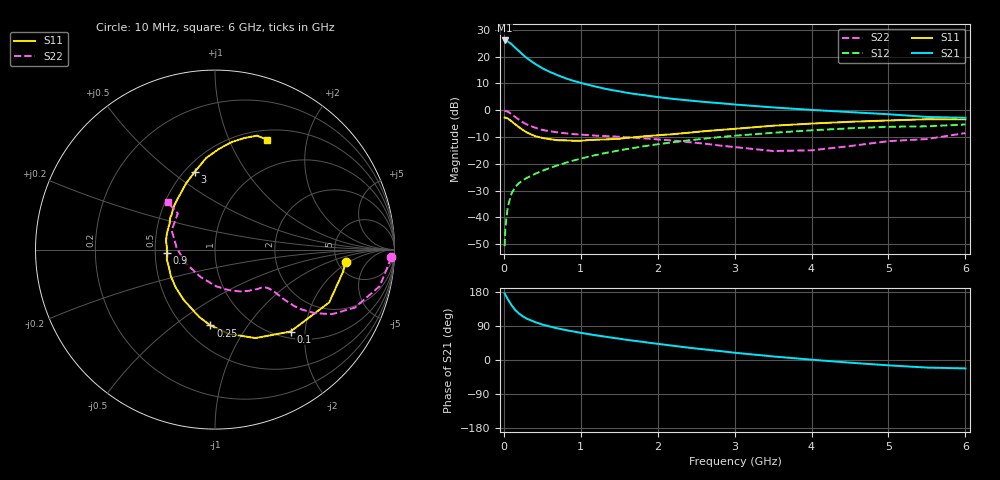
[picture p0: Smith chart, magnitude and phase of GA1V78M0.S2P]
! Infineon Technologies  Discrete & RF Semiconductors
! BF775
! Si NPN RF Bipolar Junction Transistor in SOT23
! VCE = 1.75 V  IC = 8 mA
! Common Emitter S-Parameters:  May  1996
# GHz  S  MA  R  50
!  f  S11  S21  S12  S22
! GHz  MAG  ANG  MAG  ANG  MAG  ANG  MAG  ANG
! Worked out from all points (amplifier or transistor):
!   36 points, 10 MHz to 6 GHz, reference 50 ohm
!   highest |S21| = 26.0 dB at 10 MHz (marker M1)
!   |S21| within 3 dB of that: start of sweep to 159.2 MHz
!   unconditionally stable (mu >= 1): 594.3 MHz to 3.973 GHz; 5.424 GHz to 5.631 GHz
!   at 250 MHz: K = 0.64, MSG = 23.4 dB, |S12| = -26.1 dB
!   at 1.4 GHz: K = 1.14, MAG = 9.3 dB, |S12| = -15.6 dB
!   at 6 GHz: K = 0.99, MSG = 1.2 dB, |S12| = -5.3 dB
!   S11 on the Smith chart (normalised r, x): 10 MHz: 5.91, -1.71; 100 MHz: 1.13, -1.68; 250 MHz: 0.67, -0.69; 900 MHz: 0.58, -0.02; 3 GHz: 0.56, +0.61; 6 GHz: 0.62, +1.39
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0.01  0.7304 -5.3  19.97 176.1  0.0029 86.4  0.982 -2.5
0.02  0.7239 -9.9  19.63 172.0  0.0063 85.8  0.9694 -5.1
0.05  0.701 -24.8  19.18 160.9  0.0155 77.0  0.9404 -12.5
0.1  0.6211 -47.3  17.06 144.6  0.0279 68.8  0.8436 -22.5
0.15  0.5421 -65.4  14.53 131.5  0.0371 63.0  0.7446 -28.9
0.2  0.4765 -80.5  12.54 122.1  0.044 60.3  0.6588 -32.5
0.25  0.4236 -93.4  10.74 114.7  0.0494 58.1  0.5896 -34.6
0.3  0.385 -103.3  9.346 109.0  0.0547 58.3  0.5416 -35.5
0.4  0.3293 -122.3  7.411 100.6  0.0642 58.2  0.4735 -35.8
0.5  0.3036 -136.3  6.066 93.7  0.0738 59.2  0.4288 -35.5
0.6  0.2872 -149.0  5.152 88.2  0.0838 59.7  0.4031 -35.4
0.7  0.275 -159.1  4.487 83.5  0.0934 60.4  0.3853 -35.6
0.9  0.2686 -176.1  3.546 75.4  0.1143 60.8  0.3589 -36.3
1.1  0.277 170.1  2.965 68.4  0.1353 60.2  0.3423 -38.3
1.3  0.2835 159.4  2.539 62.1  0.1567 59.2  0.3292 -40.8
1.6  0.3058 144.6  2.111 53.2  0.1882 56.8  0.3109 -45.9
2.2  0.3562 124.6  1.621 37.6  0.2519 51.0  0.2712 -59.3
3  0.4483 104.5  1.276 19.2  0.3333 41.2  0.2048 -88.0
3.5  0.5128 95.5  1.125 9.4  0.3784 34.4  0.1728 -117.3
4.5  0.6067 81.1  0.92 -7.1  0.4587 21.0  0.2138 177.5
5.5  0.677 69.7  0.747 -20.0  0.4995 6.6  0.2891 135.9
6  0.6771 64.6  0.72 -22.2  0.5404 2.6  0.3736 134.9
